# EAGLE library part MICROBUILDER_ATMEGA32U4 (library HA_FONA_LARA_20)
http://www.ladyada.net/library/eagle
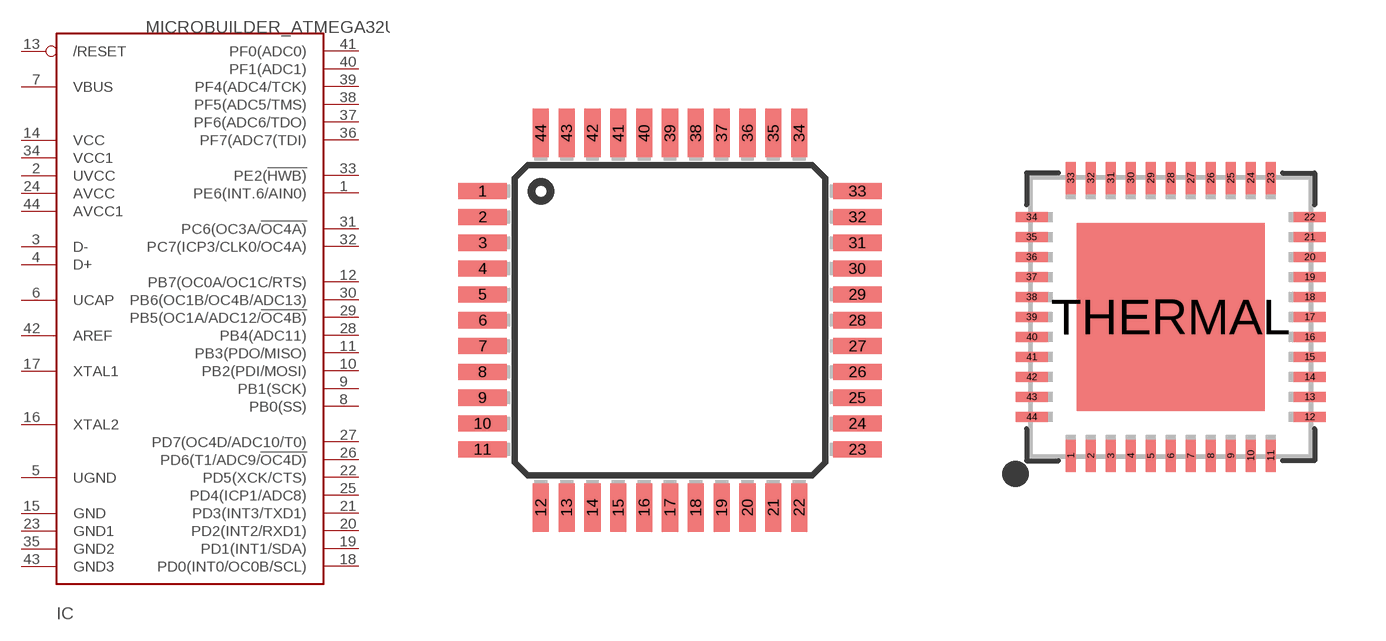
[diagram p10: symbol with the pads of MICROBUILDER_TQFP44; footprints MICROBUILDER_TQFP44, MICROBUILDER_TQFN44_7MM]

Designator prefix IC

## MICROBUILDER_ATMEGA32U4-AU  [MICROBUILDER_TQFP44]
1  PE6(INT.6/AIN0)
2  UVCC
3  D-
4  D+
5  UGND
6  UCAP
7  VBUS
8  PB0(SS)
9  PB1(SCK)
10  PB2(PDI/MOSI)
11  PB3(PDO/MISO)
12  PB7(OC0A/OC1C/RTS)
13  /RESET
14  VCC
15  GND
16  XTAL2
17  XTAL1
18  PD0(INT0/OC0B/SCL)
19  PD1(INT1/SDA)
20  PD2(INT2/RXD1)
21  PD3(INT3/TXD1)
22  PD5(XCK/CTS)
23  GND1
24  AVCC
25  PD4(ICP1/ADC8)
26  PD6(T1/ADC9/!OC4D)
27  PD7(OC4D/ADC10/T0)
28  PB4(ADC11)
29  PB5(OC1A/ADC12/!OC4B)
30  PB6(OC1B/OC4B/ADC13)
31  PC6(OC3A/!OC4A)
32  PC7(ICP3/CLK0/OC4A)
33  PE2(!HWB)
34  VCC1
35  GND2
36  PF7(ADC7(TDI)
37  PF6(ADC6/TDO)
38  PF5(ADC5/TMS)
39  PF4(ADC4/TCK)
40  PF1(ADC1)
41  PF0(ADC0)
42  AREF
43  GND3
44  AVCC1

## MICROBUILDER_ATMEGA32U4-MU  [MICROBUILDER_TQFN44_7MM]
Pads as for MICROBUILDER_TQFP44

## Footprint MICROBUILDER_TQFP44 (pad centres in mm)
smd 1.5 x 0.5: 1 -5.8,4; 2 -5.8,3.2; 3 -5.8,2.4; 4 -5.8,1.6; 5 -5.8,0.8; 6 -5.8,0; 7 -5.8,-0.8; 8 -5.8,-1.6; 9 -5.8,-2.4; 10 -5.8,-3.2; 11 -5.8,-4; 23 5.8,-4; 24 5.8,-3.2; 25 5.8,-2.4; 26 5.8,-1.6; 27 5.8,-0.8; 28 5.8,0; 29 5.8,0.8; 30 5.8,1.6; 31 5.8,2.4; 32 5.8,3.2; 33 5.8,4
smd 0.5 x 1.5: 12 -4,-5.8; 13 -3.2,-5.8; 14 -2.4,-5.8; 15 -1.6,-5.8; 16 -0.8,-5.8; 17 0,-5.8; 18 0.8,-5.8; 19 1.6,-5.8; 20 2.4,-5.8; 21 3.2,-5.8; 22 4,-5.8; 34 4,5.8; 35 3.2,5.8; 36 2.4,5.8; 37 1.6,5.8; 38 0.8,5.8; 39 0,5.8; 40 -0.8,5.8; 41 -1.6,5.8; 42 -2.4,5.8; 43 -3.2,5.8; 44 -4,5.8

## Footprint MICROBUILDER_TQFN44_7MM (pad centres in mm)
Source: http://datasheets.maxim-ic.com/en/ds/MAX9744.pdf
smd 0.25 x 0.8: 1 -2.5,-3.475; 2 -2,-3.475; 3 -1.5,-3.475; 4 -1,-3.475; 5 -0.5,-3.475; 6 0,-3.475; 7 0.5,-3.475; 8 1,-3.475; 9 1.5,-3.475; 10 2,-3.475; 11 2.5,-3.475; 23 2.5,3.475; 24 2,3.475; 25 1.5,3.475; 26 1,3.475; 27 0.5,3.475; 28 0,3.475; 29 -0.5,3.475; 30 -1,3.475; 31 -1.5,3.475; 32 -2,3.475; 33 -2.5,3.475
smd 0.8 x 0.25: 12 3.475,-2.5; 13 3.475,-2; 14 3.475,-1.5; 15 3.475,-1; 16 3.475,-0.5; 17 3.475,0; 18 3.475,0.5; 19 3.475,1; 20 3.475,1.5; 21 3.475,2; 22 3.475,2.5; 34 -3.475,2.5; 35 -3.475,2; 36 -3.475,1.5; 37 -3.475,1; 38 -3.475,0.5; 39 -3.475,0; 40 -3.475,-0.5; 41 -3.475,-1; 42 -3.475,-1.5; 43 -3.475,-2; 44 -3.475,-2.5
smd 4.7 x 4.7: THERMAL 0,0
